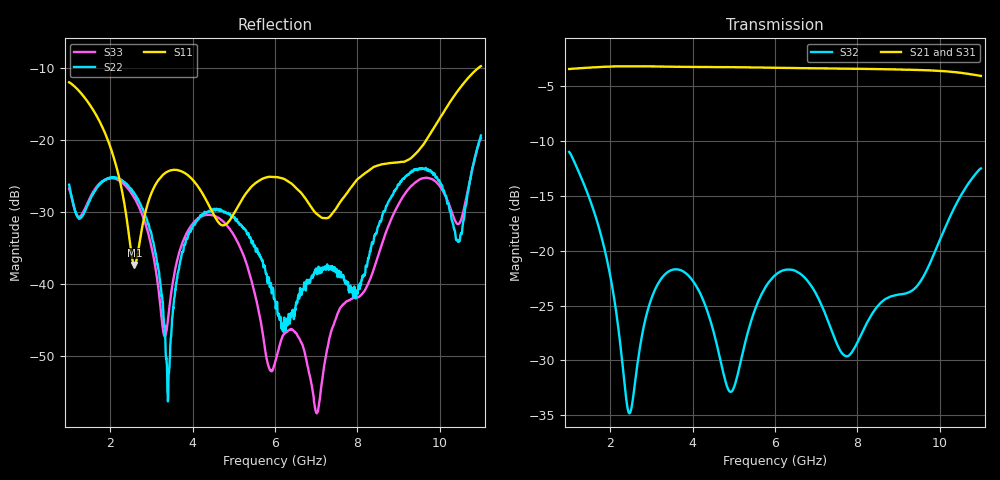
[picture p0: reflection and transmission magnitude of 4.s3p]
!The following data was pulled from an Agilent PNA
!This sNp file was generated from the data in the RF Test software
!NOTE:  Smoothing/Math/Corrections applied on any given trace ARE included in the data saved here
# MHz S dB R 50
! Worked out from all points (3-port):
!   1601 points, 1 GHz to 11 GHz, reference 50 ohm
!   strongest paths, dB at 1 GHz, 3.5 GHz, 6 GHz, 8.5 GHz, 11 GHz:
!     S21: -3.4, -3.2, -3.3, -3.4, -4.1
!     S31: -3.4, -3.2, -3.3, -3.4, -4.1
!     S32: -11.0, -21.7, -22.2, -25.0, -12.5
!   lowest |S11| = -37.4 dB at 2.587 GHz (marker M1), VSWR 1.03, Z = 49 + j0.86 ohm
!   |S11| at or under -10 dB: start of sweep to 10.94 GHz
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1000  -12.02 131.0  -3.42 -64.6  -3.42 -63.9
      -3.42 -63.7  -26.25 13.7  -11.00 -87.8
      -3.42 -63.9  -10.99 -87.8  -26.81 9.1
2587.5  -37.40 139.4  -3.17 -169.2  -3.16 -169.6
        -3.17 -169.2  -27.47 129.5  -32.45 -56.6
        -3.16 -169.7  -32.43 -56.7  -28.10 127.5
3400  -24.39 -179.4  -3.21 136.3  -3.21 135.7
      -3.21 136.3  -56.35 168.9  -21.94 -70.6
      -3.20 135.7  -21.93 -70.7  -44.97 -56.5
4268.75  -27.76 161.4  -3.24 77.8  -3.24 77.1
         -3.24 77.8  -30.28 -178.6  -24.64 -114.7
         -3.24 77.1  -24.63 -114.6  -30.52 -158.8
6000  -25.17 -148.9  -3.31 -40.8  -3.31 -41.9
      -3.31 -40.8  -42.27 79.3  -22.24 -81.9
      -3.31 -41.9  -22.24 -81.9  -51.01 -38.8
7018.75  -30.33 -142.5  -3.36 -112.0  -3.37 -113.2
         -3.36 -112.0  -38.63 103.7  -24.10 -130.5
         -3.37 -113.2  -24.08 -130.5  -57.96 -72.9
7962.5  -25.74 -94.8  -3.41 -179.1  -3.42 179.5
        -3.41 -179.2  -41.96 95.0  -28.66 -100.8
        -3.41 179.5  -28.66 -100.9  -41.92 -99.2
9325  -22.43 -84.0  -3.50 81.4  -3.52 79.8
      -3.50 81.4  -24.29 61.6  -23.64 -104.0
      -3.52 79.8  -23.65 -103.8  -26.33 60.7
10443.75  -13.16 -83.6  -3.74 -3.3  -3.77 -5.1
          -3.74 -3.3  -34.12 -93.4  -15.44 -114.2
          -3.77 -5.1  -15.44 -114.2  -31.72 -97.2
11000  -9.77 -107.6  -4.05 -44.8  -4.09 -47.8
       -4.06 -45.8  -19.40 141.4  -12.50 -141.2
       -4.09 -47.9  -12.49 -141.2  -19.81 142.9
